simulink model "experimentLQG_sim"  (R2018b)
settings: Solver=ode4  StartTime=0.0  StopTime=inf  FixedStep=1e-3  RelTol=1e-3
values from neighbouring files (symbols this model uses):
  K = lqr(sysd, Q, R)    [mainSkript_LQGexperiment.m]    (also in mainSkript_LQGexperiment_integral.m; makeFBL.m = [0; -d_2*g*sin(th_1); -d_3*g*sin(th_2)]; mainSkript_simulaceLQG.m = lqr(sysd, Qk, Rk); mainSkript_pocitaniTVLQR_simplified.m = zeros(N + 1, n_sts))
  Ts = 1e-3    (= 0.001)    [mainSkript_LQGexperiment.m]    (also in mainSkript_LQGexperiment_integral.m; mainSkript_rovniceSystemu.m; mainSkript_simulaceLQG.m; mainSkript_modifikaceParametru.m)
undefined symbols (not defined in the file or in its folder): DiscIntNeverNeededParam, Humusoft, MF624
libraries: sldrtlib x8, simulink x6, sharedTrackingLibrary x1

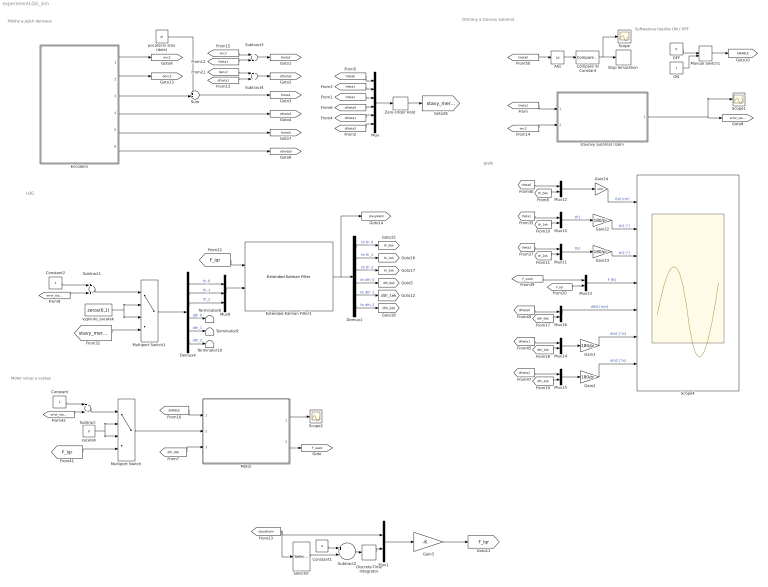
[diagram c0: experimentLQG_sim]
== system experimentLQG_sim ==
  note: Polohy a jejich derivace
  note: Softwarove tlacitko ON / OFF
  note: Ochrany a stavovy automat
  note: Motor vstup a vystup
  note: LQG
  note: grafy
  Abs : Abs
  Compare To Constant : simulink/Logic and Bit Operations/Compare To Constant  relop=>  const=0.5  OutDataTypeStr=boolean
  Constant : Constant
  Constant1 : Constant  Value=0
  Constant2 : Constant
  Demux1 : Demux  Outputs=6
  Demux4 : Demux  Outputs=6
  Discrete-Time Integrator : DiscreteIntegrator  SampleTime=Ts  ICPrevOutput=DiscIntNeverNeededParam  ICPrevScaledInput=DiscIntNeverNeededParam
  Encoders : Subsystem
  Extended Kalman Filter1 : sharedTrackingLibrary/Extended Kalman Filter  StateTransitionFcn=nonLinKalmFcn_pn0  HasStateTransitionJacobianFcn=on  StateTransitionJacobianFcn=countJacobDIP_pn0  HasAdditiveProcessNoise=Additive  ProcessNoise=Q_kalm  HasTimeVaryingProcessNoise=off  HasStateTransitionFcnExtraArgument=1  InitialState=q_0  InitialStateCovariance=1e-3*eye(6)  MeasurementFcn1=mereniStavuKalm  HasMeasurementJacobianFcn1=off  HasMeasurementEnablePort1=off  HasAdditiveMeasurementNoise1=Additive  MeasurementNoise1=R_kalm  HasTimeVaryingMeasurementNoise1=off  HasMeasurementFcnExtraArgument1=0  MeasurementFcn2=myMeasurementFcn  HasMeasurementJacobianFcn2=off  HasMeasurementEnablePort2=off  HasAdditiveMeasurementNoise2=Additive  MeasurementNoise2=1  HasTimeVaryingMeasurementNoise2=off  HasMeasurementFcnExtraArgument2=0  MeasurementFcn3=myMeasurementFcn  HasMeasurementJacobianFcn3=off  HasMeasurementEnablePort3=off  HasAdditiveMeasurementNoise3=Additive  MeasurementNoise3=1  HasTimeVaryingMeasurementNoise3=off  HasMeasurementFcnExtraArgument3=0  MeasurementFcn4=myMeasurementFcn  HasMeasurementJacobianFcn4=off  HasMeasurementEnablePort4=off  HasAdditiveMeasurementNoise4=Additive  MeasurementNoise4=1  HasTimeVaryingMeasurementNoise4=off  HasMeasurementFcnExtraArgument4=0  MeasurementFcn5=myMeasurementFcn  HasMeasurementJacobianFcn5=off  HasMeasurementEnablePort5=off  HasAdditiveMeasurementNoise5=Additive  MeasurementNoise5=1  HasTimeVaryingMeasurementNoise5=off  HasMeasurementFcnExtraArgument5=0  EnableMultirate=off  StateTransitionFcnSampleTime=1  MeasurementFcn1SampleTime=1  MeasurementFcn2SampleTime=1  MeasurementFcn3SampleTime=1  MeasurementFcn4SampleTime=1  MeasurementFcn5SampleTime=1  UseCurrentEstimator=on  OutputStateCovariance=off  DataType=double  SampleTime=1e-3  NumberOfMeasurements=1
  Gain{1..2,22..23} (4 alike) : Gain  Gain=180/pi
  Gain24 : Gain  Gain=100
  Gain3 : Gain  Gain=-K  Multiplication=Matrix(K*u) (u vector)
  Manual Switch1 : ManualSwitch  CurrentSetting=0
  Motor : Subsystem
  Multiport Switch : MultiPortSwitch
  Multiport Switch1 : MultiPortSwitch
  Mux : Mux  Inputs=6
  Mux{1,10..16} (8 alike) : Mux  Inputs=2
  Mux9 : Mux  Inputs=3
  OFF : Constant  Value=0
  ON : Constant
  Scope : Scope
  Scope1 : Scope
  Scope2 : Scope
  Scope4 : Scope  NumInputPorts=7
  Selector : Selector  InputPortWidth=6  IndexOptions=Index vector (dialog)  Indices=[1]  OutputSizes=1
  Stop Simulation : Stop
  Subtract{,1,3..4} (4 alike) : Sum
  Subtract2 : Sum  Inputs=+-
  Sum : Sum  Inputs=++|
  Terminator10 : Terminator
  Terminator8 : Terminator
  Terminator9 : Terminator
  Zero-Order Hold : ZeroOrderHold  SampleTime=1e-3
  pocatecni stav (dole) : Constant  Value=pi
  stavovy automat rizeni : Subsystem
  vypnuto_zacatek : Constant  Value=zeros(6,1)
  zacatek : Constant  Value=0
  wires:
  [theta1] -> stavovy automat rizeni/1(theta1)
  stavovy automat rizeni/1(error_state) -> Scope1/1, [error_state]
  Encoders/6(v [m/s]) -> [dtheta0]
  Encoders/5(x [m]) -> [theta0]
  Demux4/5 -> Terminator9/1  "dth_1"
  Demux4/1 -> Mux9/1  "th_0"
  Demux4/6 -> Terminator10/1  "dth_2"
  Demux4/4 -> Terminator8/1  "dth_0"
  Demux4/3 -> Mux9/3  "th_2"
  Demux4/2 -> Mux9/2  "th_1"
  [dtheta2] -> Mux/6
  [theta1] -> Mux/2
  [theta2] -> Mux/3
  [dtheta1] -> Mux/5
  [theta0] -> Mux/1
  [dtheta0] -> Mux/4
  Mux13/1 -> Scope4/4  "F [N]"
  [theta1] -> Mux10/1
  Mux12/1 -> Gain24/1
  Gain23/1 -> Scope4/3  "th2 [°]"
  [theta2] -> Mux11/1
  Mux11/1 -> Gain23/1  "th2"
  [theta0] -> Mux12/1
  [th_1ek] -> Mux10/2
  Gain24/1 -> Scope4/1  "th0 [cm]"
  Mux10/1 -> Gain22/1  "th1"
  Gain22/1 -> Scope4/2  "th1 [°]"
  [enc2] -> stavovy automat rizeni/2(enc2)
  [error_state] -> Subtract/2
  Subtract/1 -> Multiport Switch/1
  Constant/1 -> Subtract/1
  [dtheta1] -> Mux14/1
  [dtheta0] -> Mux16/1
  Mux15/1 -> Gain2/1
  [dtheta2] -> Mux15/1
  Mux16/1 -> Scope4/5  "dth0 [m/s]"
  Mux14/1 -> Gain1/1
  OFF/1 -> Manual Switch1/1
  ON/1 -> Manual Switch1/2
  Abs/1 -> Compare To Constant/1
  [theta0] -> Abs/1
  Compare To Constant/1 -> Scope/1, Stop Simulation/1
  Manual Switch1/1 -> [ENABLE]
  vypnuto_zacatek/1 -> Multiport Switch1/3, Multiport Switch1/2
  Constant2/1 -> Subtract1/1
  [error_state] -> Subtract1/2
  Subtract1/1 -> Multiport Switch1/1
  Multiport Switch1/1 -> Demux4/1
  zacatek/1 -> Multiport Switch/3, Multiport Switch/2
  [stavy_merene] -> Multiport Switch1/4
  Gain1/1 -> Scope4/6  "dth1 [°/s]"
  Gain2/1 -> Scope4/7  "dth2 [°/s]"
  Subtract3/1 -> [theta2]
  Encoders/1(enc2 [rad]) -> [enc2]
  Subtract4/1 -> [dtheta2]
  Encoders/4(dth1 [rad/s]) -> [dtheta1]
  [theta1] -> Subtract3/2
  [dtheta1] -> Subtract4/2
  Sum/1 -> [theta1]
  Encoders/3(th1 [rad]) -> Sum/2
  pocatecni stav (dole)/1 -> Sum/1
  [dth_0ek] -> Motor/3(v [m/s])
  [ENABLE] -> Motor/1(ENABLE)
  Multiport Switch/1 -> Motor/2(F_in [N])
  Motor/1(sat_flag) -> Scope2/1
  Demux1/3 -> [th_2ek]  "lin th_2"
  Demux1/2 -> [th_1ek]  "lin th_1"
  Demux1/4 -> [dth_0ek]  "lin dth_0"
  Demux1/5 -> [dth_1ek]  "lin dth_1"
  Demux1/1 -> [th_0ek]  "lin th_0"
  Extended Kalman Filter1/1 -> [stavyKalm], Demux1/1
  Demux1/6 -> [dth_2ek]  "lin dth_2"
  [th_0ek] -> Mux12/2
  [th_2ek] -> Mux11/2
  [dth_0ek] -> Mux16/2
  [dth_1ek] -> Mux14/2
  [F_lqr] -> Mux13/2
  [F_used] -> Mux13/1
  [F_lqr] -> Multiport Switch/4
  Mux/1 -> Zero-Order Hold/1
  [dth_2ek] -> Mux15/2
  Mux9/1 -> Extended Kalman Filter1/2
  Zero-Order Hold/1 -> [stavy_merene]
  [enc2] -> Subtract3/1
  Encoders/2(denc2 [rad/s]) -> [denc2]
  [denc2] -> Subtract4/1
  Motor/2(F_used [N]) -> [F_used]
  [F_lqr] -> Extended Kalman Filter1/1
  [stavyKalm] -> Selector/1, Mux1/1
  Mux1/1 -> Gain3/1
  Discrete-Time Integrator/1 -> Mux1/2
  Subtract2/1 -> Discrete-Time Integrator/1
  Gain3/1 -> [F_lqr]
  Selector/1 -> Subtract2/2
  Constant1/1 -> Subtract2/1

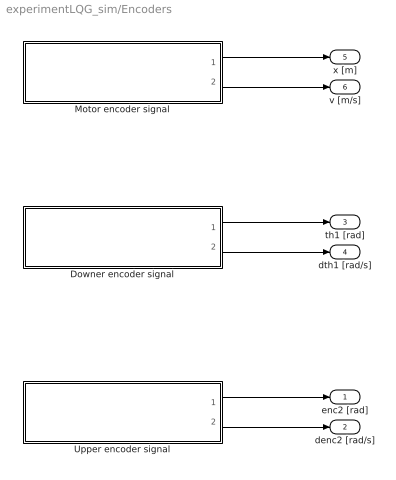
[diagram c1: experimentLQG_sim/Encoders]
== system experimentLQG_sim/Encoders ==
  Downer encoder signal : Subsystem
  Motor encoder signal : Subsystem
  Upper encoder signal : Subsystem
  enc2 [rad] : Outport
  denc2 [rad/s] : Outport  Port=2
  th1 [rad] : Outport  Port=3
  dth1 [rad/s] : Outport  Port=4
  x [m] : Outport  Port=5
  v [m/s] : Outport  Port=6
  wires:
  Downer encoder signal/2(omega [rad/s]) -> dth1 [rad/s]/1
  Downer encoder signal/1(phi [rad]) -> th1 [rad]/1
  Motor encoder signal/1(x [m]) -> x [m]/1
  Motor encoder signal/2(v [m/s]) -> v [m/s]/1
  Upper encoder signal/2(omega [rad/s]) -> denc2 [rad/s]/1
  Upper encoder signal/1(phi [rad]) -> enc2 [rad]/1

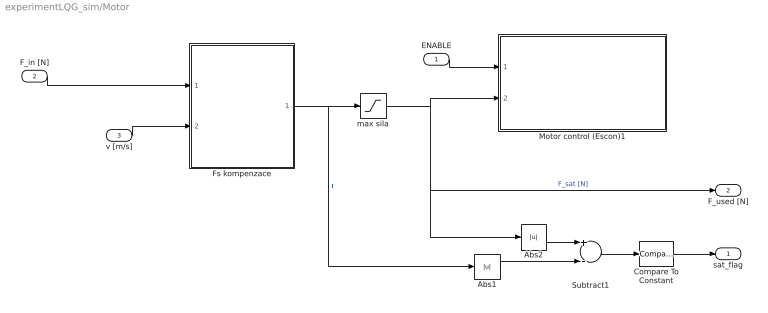
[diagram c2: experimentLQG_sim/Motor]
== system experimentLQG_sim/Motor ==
  ENABLE : Inport
  F_in [N] : Inport  Port=2
  v [m/s] : Inport  Port=3
  Abs1 : Abs
  Abs2 : Abs
  Compare To Constant : simulink/Logic and Bit Operations/Compare To Constant  relop=>  const=1e-8  OutDataTypeStr=boolean
  Fs kompenzace : Subsystem
  Motor control (Escon)1 : Subsystem
  Subtract1 : Sum  Inputs=+-
  max sila : Saturate  UpperLimit=40  LowerLimit=-40
  sat_flag : Outport
  F_used [N] : Outport  Port=2
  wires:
  ENABLE/1 -> Motor control (Escon)1/1(ENABLE)
  v [m/s]/1 -> Fs kompenzace/2(v [m/s])
  F_in [N]/1 -> Fs kompenzace/1(F_in [N])
  Compare To Constant/1 -> sat_flag/1
  Subtract1/1 -> Compare To Constant/1
  Abs1/1 -> Subtract1/2
  max sila/1 -> Motor control (Escon)1/2(Ref strength [N]), F_used [N]/1, Abs2/1  "F_sat [N]"
  Abs2/1 -> Subtract1/1
  Fs kompenzace/1(F_out [N]) -> max sila/1, Abs1/1  "F"

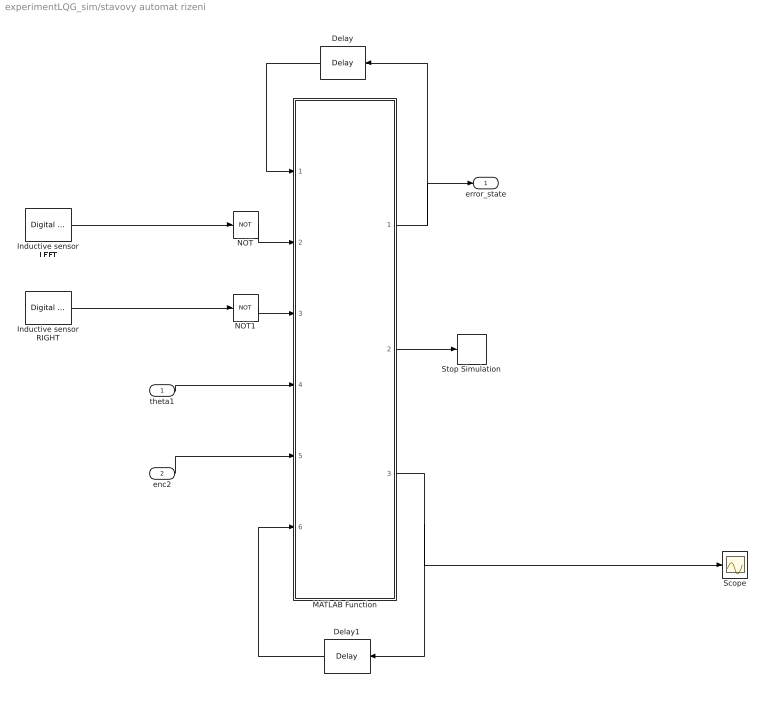
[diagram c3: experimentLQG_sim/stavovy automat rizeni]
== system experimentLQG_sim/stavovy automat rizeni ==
  theta1 : Inport
  enc2 : Inport  Port=2
  Delay : Delay  DelayLength=1  InitialCondition=0  UseCircularBuffer=on
  Delay1 : Delay  DelayLength=1  InitialCondition=0  UseCircularBuffer=on
  Inductive sensor LEFT : sldrtlib/Digital Input  SampleTime=0.001  MaxMissedTicks=1e6  ShowMissedTicks=off  YieldWhenWaiting=off  DrvName=Humusoft/MF624  DrvAddress=4294967295  DrvOptions=0  Channels=1  BitMode=1  DataType=1
  Inductive sensor RIGHT : sldrtlib/Digital Input  SampleTime=0.001  MaxMissedTicks=1e6  ShowMissedTicks=off  YieldWhenWaiting=off  DrvName=Humusoft/MF624  DrvAddress=4294967295  DrvOptions=0  Channels=2  BitMode=1  DataType=1
  MATLAB Function : MATLAB Function  TreatAsAtomicUnit=on
  NOT : Logic  Operator=NOT  IconShape=distinctive  AllPortsSameDT=off  OutDataTypeStr=boolean
  NOT1 : Logic  Operator=NOT  IconShape=distinctive  AllPortsSameDT=off  OutDataTypeStr=boolean
  Scope : Scope
  Stop Simulation : Stop
  error_state : Outport
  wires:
  theta1/1 -> MATLAB Function/4(theta1)
  Inductive sensor LEFT/1 -> NOT/1
  NOT/1 -> MATLAB Function/2(leftSens)
  NOT1/1 -> MATLAB Function/3(rightSens)
  Inductive sensor RIGHT/1 -> NOT1/1
  MATLAB Function/1(err_state) -> Delay/1, error_state/1
  MATLAB Function/2(total_err) -> Stop Simulation/1
  Delay/1 -> MATLAB Function/1(last_err_state)
  enc2/1 -> MATLAB Function/5(enc2)
  MATLAB Function/3(count) -> Delay1/1, Scope/1
  Delay1/1 -> MATLAB Function/6(last_count)

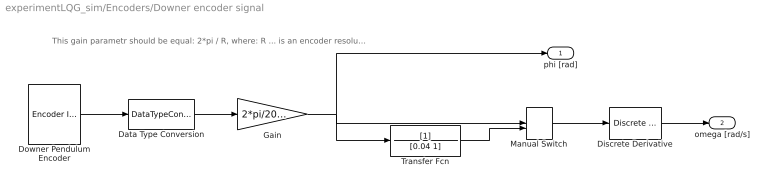
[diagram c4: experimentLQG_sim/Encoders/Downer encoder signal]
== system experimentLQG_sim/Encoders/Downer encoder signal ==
  note: This gain parametr should be equal: 2*pi / R, where: R ... is an encoder resolution
  Data Type Conversion : DataTypeConversion  OutDataTypeStr=double
  Discrete Derivative : simulink/Discrete/Discrete Derivative  gainval=1.0  ICPrevScaledInput=0.0  OutMin=[]  OutMax=[]  OutDataType=fixdt(1, 16)  OutScaling=2^-10  DoSatur=off
  Downer Pendulum Encoder : sldrtlib/Encoder Input  SampleTime=0.001  MaxMissedTicks=1e8  ShowMissedTicks=off  YieldWhenWaiting=off  DrvName=Humusoft/MF624  DrvAddress=4294967295  DrvOptions=0  Channels=2  QuadMode=3  IndexPulse=1  InputFilter=Inf  DataType=7
  Gain : Gain  Gain=2*pi/2048
  Manual Switch : ManualSwitch  CurrentSetting=0
  Transfer Fcn : TransferFcn  Denominator=[0.04 1]
  phi [rad] : Outport
  omega [rad/s] : Outport  Port=2
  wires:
  Downer Pendulum Encoder/1 -> Data Type Conversion/1
  Discrete Derivative/1 -> omega [rad/s]/1
  Data Type Conversion/1 -> Gain/1
  Gain/1 -> Transfer Fcn/1, Manual Switch/1, phi [rad]/1
  Manual Switch/1 -> Discrete Derivative/1
  Transfer Fcn/1 -> Manual Switch/2

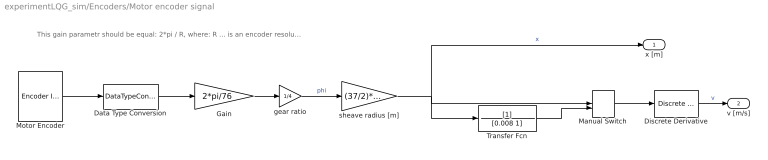
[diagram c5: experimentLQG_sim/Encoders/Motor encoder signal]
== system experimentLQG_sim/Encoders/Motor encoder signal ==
  note: This gain parametr should be equal: 2*pi / R, where: R ... is an encoder resolution
  Data Type Conversion : DataTypeConversion  OutDataTypeStr=double
  Discrete Derivative : simulink/Discrete/Discrete Derivative  gainval=1.0  ICPrevScaledInput=0.0  OutMin=[]  OutMax=[]  OutDataType=fixdt(1, 16)  OutScaling=2^-10  DoSatur=off
  Gain : Gain  Gain=2*pi/76
  Manual Switch : ManualSwitch  CurrentSetting=0
  Motor Encoder : sldrtlib/Encoder Input  SampleTime=0.001  MaxMissedTicks=1e8  ShowMissedTicks=off  YieldWhenWaiting=off  DrvName=Humusoft/MF624  DrvAddress=4294967295  DrvOptions=0  Channels=3  QuadMode=3  IndexPulse=1  InputFilter=Inf  DataType=7
  Transfer Fcn : TransferFcn  Denominator=[0.008 1]
  gear ratio : Gain  Gain=1/4
  sheave radius [m] : Gain  Gain=(37/2)*1e-3
  x [m] : Outport
  v [m/s] : Outport  Port=2
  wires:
  Motor Encoder/1 -> Data Type Conversion/1
  Discrete Derivative/1 -> v [m/s]/1  "v"
  Data Type Conversion/1 -> Gain/1
  Gain/1 -> gear ratio/1
  sheave radius [m]/1 -> Transfer Fcn/1, Manual Switch/1, x [m]/1  "x"
  gear ratio/1 -> sheave radius [m]/1  "phi"
  Transfer Fcn/1 -> Manual Switch/2
  Manual Switch/1 -> Discrete Derivative/1

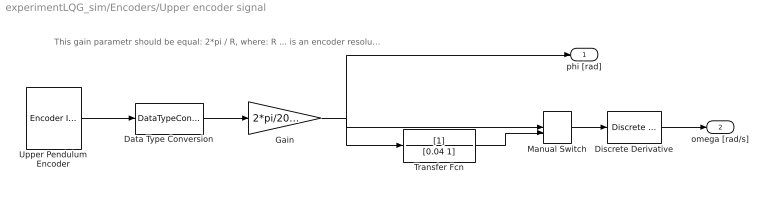
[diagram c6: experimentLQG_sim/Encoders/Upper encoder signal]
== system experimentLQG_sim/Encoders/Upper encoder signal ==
  note: This gain parametr should be equal: 2*pi / R, where: R ... is an encoder resolution
  Data Type Conversion : DataTypeConversion  OutDataTypeStr=double
  Discrete Derivative : simulink/Discrete/Discrete Derivative  gainval=1.0  ICPrevScaledInput=0.0  OutMin=[]  OutMax=[]  OutDataType=fixdt(1, 16)  OutScaling=2^-10  DoSatur=off
  Gain : Gain  Gain=2*pi/2048
  Manual Switch : ManualSwitch  CurrentSetting=0
  Transfer Fcn : TransferFcn  Denominator=[0.04 1]
  Upper Pendulum Encoder : sldrtlib/Encoder Input  SampleTime=0.001  MaxMissedTicks=1e8  ShowMissedTicks=off  YieldWhenWaiting=off  DrvName=Humusoft/MF624  DrvAddress=4294967295  DrvOptions=0  Channels=4  QuadMode=3  IndexPulse=1  InputFilter=Inf  DataType=7
  phi [rad] : Outport
  omega [rad/s] : Outport  Port=2
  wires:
  Upper Pendulum Encoder/1 -> Data Type Conversion/1
  Discrete Derivative/1 -> omega [rad/s]/1
  Data Type Conversion/1 -> Gain/1
  Manual Switch/1 -> Discrete Derivative/1
  Transfer Fcn/1 -> Manual Switch/2
  Gain/1 -> Manual Switch/1, Transfer Fcn/1, phi [rad]/1

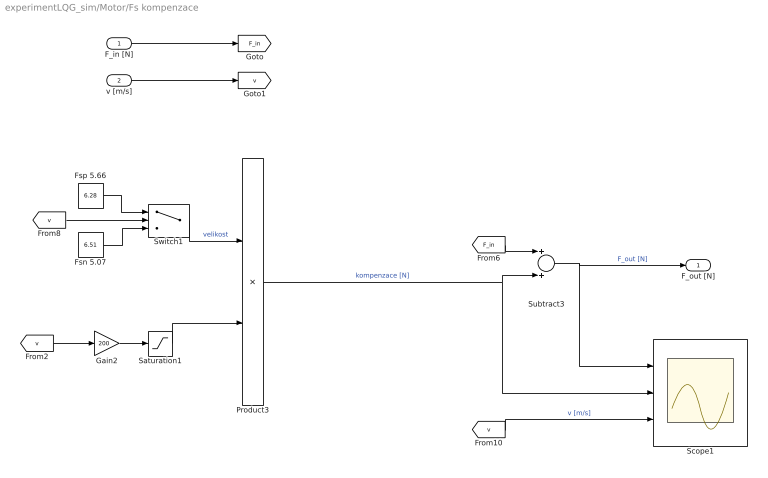
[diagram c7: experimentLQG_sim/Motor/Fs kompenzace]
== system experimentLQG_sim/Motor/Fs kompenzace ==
  F_in [N] : Inport
  v [m/s] : Inport  Port=2
  Fsn 5.07 : Constant  Value=6.51
  Fsp 5.66 : Constant  Value=6.28
  Gain2 : Gain  Gain=200
  Product3 : Product
  Saturation1 : Saturate  UpperLimit=1  LowerLimit=-1
  Scope1 : Scope  NumInputPorts=3
  Subtract3 : Sum
  Switch1 : Switch
  F_out [N] : Outport
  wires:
  F_in [N]/1 -> [F_in]
  v [m/s]/1 -> [v]
  Fsn 5.07/1 -> Switch1/3
  [v] -> Switch1/2
  Fsp 5.66/1 -> Switch1/1
  [F_in] -> Subtract3/1
  [v] -> Scope1/3  "v [m/s]"
  Subtract3/1 -> F_out [N]/1, Scope1/1  "F_out [N]"
  Switch1/1 -> Product3/1  "velikost"
  Product3/1 -> Subtract3/2, Scope1/2  "kompenzace [N]"
  Saturation1/1 -> Product3/2
  [v] -> Gain2/1
  Gain2/1 -> Saturation1/1

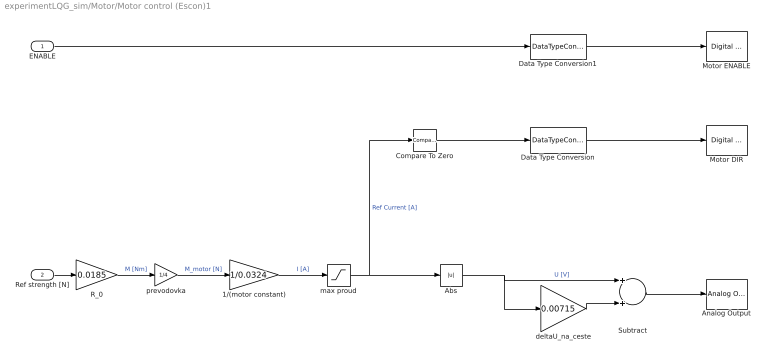
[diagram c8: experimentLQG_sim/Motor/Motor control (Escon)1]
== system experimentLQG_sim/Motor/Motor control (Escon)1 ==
  ENABLE : Inport
  Ref strength [N] : Inport  Port=2
  1/(motor constant) : Gain  Gain=1/0.0324
  Abs : Abs
  Analog Output : sldrtlib/Analog Output  SampleTime=Ts  MaxMissedTicks=1e6  ShowMissedTicks=off  YieldWhenWaiting=off  DrvName=Humusoft/MF624  DrvAddress=4294967295  DrvOptions=0  Channels=6  RangeMode=1  VoltRange=1  InitialValue=0  FinalValue=0
  Compare To Zero : simulink/Logic and Bit Operations/Compare To Zero  relop=>=  OutDataTypeStr=boolean
  Data Type Conversion : DataTypeConversion  OutDataTypeStr=boolean
  Data Type Conversion1 : DataTypeConversion  OutDataTypeStr=boolean
  Motor DIR : sldrtlib/Digital Output  SampleTime=Ts  MaxMissedTicks=1e6  ShowMissedTicks=off  YieldWhenWaiting=off  DrvName=Humusoft/MF624  DrvAddress=4294967295  DrvOptions=0  Channels=5  BitMode=1  InitialValue=0  FinalValue=0
  Motor ENABLE : sldrtlib/Digital Output  SampleTime=Ts  MaxMissedTicks=1e6  ShowMissedTicks=off  YieldWhenWaiting=off  DrvName=Humusoft/MF624  DrvAddress=4294967295  DrvOptions=0  Channels=2  BitMode=1  InitialValue=0  FinalValue=0
  R_0 : Gain  Gain=0.0185
  Subtract : Sum
  deltaU_na_ceste : Gain  Gain=0.00715
  max proud : Saturate  UpperLimit=7.5  LowerLimit=-7.5
  prevodovka : Gain  Gain=1/4
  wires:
  Abs/1 -> deltaU_na_ceste/1, Subtract/1  "U [V]"
  deltaU_na_ceste/1 -> Subtract/2
  Subtract/1 -> Analog Output/1
  Data Type Conversion/1 -> Motor DIR/1
  prevodovka/1 -> 1/(motor constant)/1  "M_motor [N]"
  R_0/1 -> prevodovka/1  "M [Nm]"
  ENABLE/1 -> Data Type Conversion1/1
  Ref strength [N]/1 -> R_0/1
  max proud/1 -> Compare To Zero/1, Abs/1  "Ref Current [A]"
  1/(motor constant)/1 -> max proud/1  "I [A]"
  Data Type Conversion1/1 -> Motor ENABLE/1
  Compare To Zero/1 -> Data Type Conversion/1

== matlab function experimentLQG_sim/stavovy 
automat rizeni/MATLAB Function ==
function [err_state, total_err, count] = fcn(last_err_state, leftSens, rightSens, theta1, enc2, last_count)

err_state = last_err_state; % pokud zadna zmena v erroru, tak zadna zmena v instrukcich
total_err  = 0; % nevypinat
stab_prah = 2; % interval horni pozice [°]
konec_stab = 25; % konec stabilizace [°]

count = last_count + 1;

switch(err_state)
    
    case 0 % zacatek (ceka se na zvednuti kyvadla)
        if (abs(theta1) <= deg2rad(stab_prah)) && (abs(enc2) <= deg2rad(stab_prah))
            count = 0;
            err_state = 1; % jde se stabilizovat?
        end
        
    case 1 % kyvadlo nahore, cekat
        
        if ~((abs(theta1) <= deg2rad(stab_prah)) && (abs(enc2) <= deg2rad(stab_prah)))
            err_state = 0;
            
        elseif count > 200 % cekat 0.2 s
            err_state = 2; % jde se stabilizovat!
        end
        
    case 2 % kyvadlo nahore, stabilizovat
        if (abs(theta1) >= deg2rad(konec_stab)) || (leftSens == 1) || (rightSens == 1) % vyjeti z kolejnice, nebo zatoceny kabel
            err_state = 100;
            total_err = 1;
        end
        
    otherwise % totalni error -> vypnout
        total_err = 1; % vypnout
        
end

end
